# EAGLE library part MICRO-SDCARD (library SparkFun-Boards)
microSD Card Footprint This is the mechnical footprint with connections for soldering a microSD card - NOT for a socket for the card. SparkFun Products: MicroSD Card with Adapter - 8 GB SparkFun microSD Sniffer
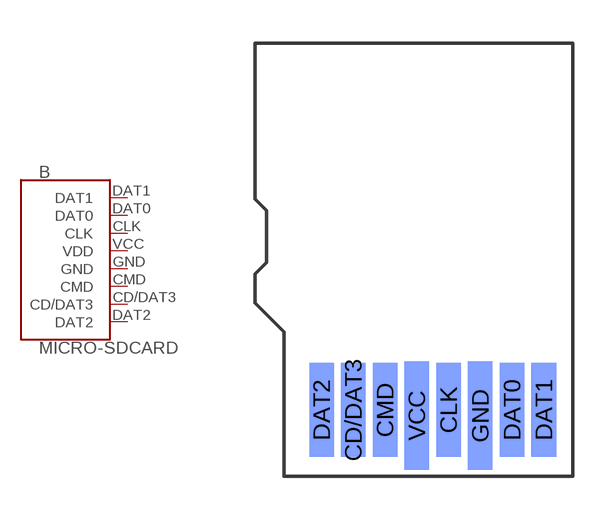
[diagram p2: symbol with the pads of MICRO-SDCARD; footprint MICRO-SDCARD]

Designator prefix B

## MICRO-SDCARD  [MICRO-SDCARD]
CD/DAT3  CD/DAT3
CLK  CLK
CMD  CMD
DAT0  DAT0
DAT1  DAT1
DAT2  DAT2
GND  GND  pwr
VCC  VDD  pwr

## Footprint MICRO-SDCARD (pad centres in mm)
microSD Card Footprint Silk outline with pads for SMD. Specifications: Pin count:8 Area:0.45x0.6 in Example device(s): MicroSD Card
smd 0.85 x 3.25 bottom: CD/DAT3 -2.52,-5.32; CLK 0.78,-5.32; CMD -1.42,-5.32; DAT0 2.98,-5.32; DAT1 4.08,-5.32; DAT2 -3.62,-5.32
smd 0.85 x 3.75 bottom: GND 1.88,-5.52; VCC -0.32,-5.52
